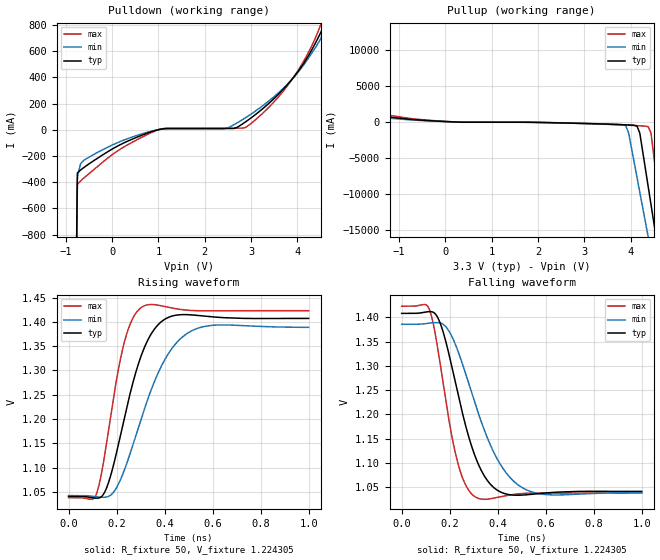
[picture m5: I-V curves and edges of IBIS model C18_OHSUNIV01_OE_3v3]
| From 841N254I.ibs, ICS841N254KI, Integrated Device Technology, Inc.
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[Model] C18_OHSUNIV01_OE_3v3
Model_type   Output
Polarity   Non-Inverting
|   typ   min   max
C_comp   2pF   1.5pF   2.5pF
Vmeas = 1.22V
Rref = 50
Cref = 0
Vref = 1.22V
|   typ   min   max
[Voltage range]   3.3V   3.135V   3.465V
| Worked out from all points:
|   slope of the pulldown table from 0 to 0.495 V, typ, clamps not added: 5.82 ohm
|   slope of the pullup table from 0 to 0.495 V, typ, clamps not added: 4.85 ohm
|   rising waveform, R_fixture 50, V_fixture 1.224305: 20-80 % time 113ps typ, 153ps min, 79.4ps max; typ from 1.04 V to 1.41 V
|   falling waveform, R_fixture 50, V_fixture 1.224305: 20-80 % time 113ps typ, 153ps min, 79.4ps max; typ from 1.41 V to 1.04 V
[Pulldown]
|Voltage   I (typ)   I (min)   I (max)
-3.3V     -100.9A    -86.69A    -124.9A
-1.26V    -16.29A    -16.38A    -16.38A
-750mV    -330.7mA   -374.2mA   -416.8mA
-679.8mV  -307.1mA   -259.2mA   -390.7mA
-559.3mV  -275.3mA   -222mA     -352.9mA
1.007V    1.155mA    1.465mA    547.5uA
2.452V    9.651mA    8.893mA    12.23mA
2.874V    58.6mA     90.38mA    16.43mA
3.777V    341.9mA    344.8mA    332.6mA
4.5V      740mA      692.6mA    799.1mA
4.928V    1.104A     1.4A       1.269A
6.6V      11.32A     11.27A     11.63A
[Pullup]
|Voltage   I (typ)   I (min)   I (max)
-3.3V     11.37A     10.32A     13.25A
-2.28V    4.031A     4.242A     3.796A
-1.77V    1.285A     1.289A     1.794A
42.99mV   98.4mA     84.71mA    114.4mA
3.898V    -352.9mA   -491.8mA   -391.6mA
3.958V    -368.4mA   -1.481A    -409.6mA
4.199V    -1.493A    -9.723A    -487.2mA
4.38V     -8.922A    -15.91A    -606.3mA
4.44V     -11.4A     -17.97A    -1.467A
4.51V     -14.29A    -20.38A    -5.143A
4.928V    -31.5A     -34.72A    -27.13A
6.6V      -100.8A    -92.33A    -115.9A
[Ramp]
|   typ   min   max
dV/dt_r   0.302/0.176n   0.284/0.236n   0.321/0.125n
dV/dt_f   0.302/0.176n   0.284/0.236n   0.321/0.125n
R_load =   50.0000
[Rising Waveform]
R_fixture = 50
V_fixture   =1.224305   |Vcc_typ
V_fixture_min=1.21395  |Vcc_min
V_fixture_max=1.230485  |Vcc_max
C_fixture = 0.0p
| Time   typ   min   max
0s        1.041V     1.042V     1.038V
116.1ps   1.037V     1.04V      1.046V
162.2ps   1.063V     1.04V      1.163V
225.2ps   1.186V     1.085V     1.344V
260.3ps   1.26V      1.135V     1.4V
300.3ps   1.327V     1.197V     1.429V
384.4ps   1.4V       1.307V     1.433V
506.5ps   1.415V     1.38V      1.424V
622.6ps   1.41V      1.394V     1.423V
1ns       1.407V     1.389V     1.423V
[Falling Waveform]
R_fixture = 50
V_fixture   =1.224305   |Vcc_typ
V_fixture_min=1.21395  |Vcc_min
V_fixture_max=1.230485  |Vcc_max
C_fixture = 0.0p
| Time   typ   min   max
0s        1.408V     1.386V     1.423V
116.1ps   1.412V     1.388V     1.415V
162.2ps   1.386V     1.388V     1.298V
225.2ps   1.262V     1.342V     1.117V
260.3ps   1.189V     1.293V     1.061V
300.3ps   1.121V     1.231V     1.032V
384.4ps   1.049V     1.121V     1.028V
506.5ps   1.034V     1.048V     1.037V
622.6ps   1.039V     1.034V     1.038V
1ns       1.041V     1.039V     1.038V
